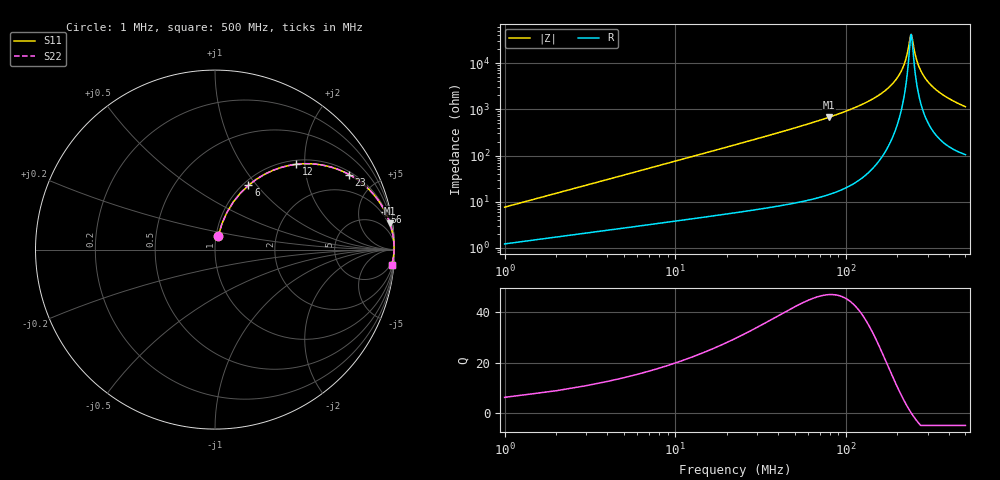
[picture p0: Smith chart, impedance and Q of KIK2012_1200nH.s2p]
!version-2
!date-01.2022
!Series
# MHz S RI R 50
!Freq ReS11 ImS11 ReS21 ImS21 ReS12 ImS12 ReS22 ImS22
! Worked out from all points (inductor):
!   500 points, 1 MHz to 500 MHz, reference 50 ohm
!   read as one part in series: L = 1.2 uH near 3 MHz
!   highest Q = 47 at 79 MHz (marker M1), where L = 1.35 uH
!   self-resonance near 240 MHz
!   S11 on the Smith chart (normalised r, x): 1 MHz: 1.02, +0.15; 6 MHz: 1.06, +0.91; 12 MHz: 1.08, +1.81; 23 MHz: 1.12, +3.50; 56 MHz: 1.20, +8.93; 500 MHz: 3, -23
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1  0.0175 0.0732  0.9825 -0.0732  0.9825 -0.0732  0.0175 0.0732
4  0.1015 0.2647  0.8985 -0.2647  0.8985 -0.2647  0.1015 0.2647
6  0.186 0.3579  0.814 -0.3579  0.814 -0.3579  0.186 0.3579
12  0.454 0.4754  0.546 -0.4754  0.546 -0.4754  0.454 0.4754
23  0.747 0.4183  0.253 -0.4183  0.253 -0.4183  0.747 0.4183
36  0.8787 0.3132  0.1213 -0.3132  0.1213 -0.3132  0.8787 0.3132
56  0.9479 0.2111  0.0521 -0.2111  0.0521 -0.2111  0.9479 0.2111
79  0.9751 0.1455  0.0249 -0.1455  0.0249 -0.1455  0.9751 0.1455
85  0.979 0.1332  0.021 -0.1332  0.021 -0.1332  0.979 0.1332
168  0.9965 0.0402  0.00348 -0.0402  0.00348 -0.0402  0.9965 0.0402
195  0.9975 0.0232  0.00251 -0.0232  0.00251 -0.0232  0.9975 0.0232
214  0.9977 0.0129  0.00229 -0.0129  0.00229 -0.0129  0.9977 0.0129
226  0.9977 0.00687  0.00228 -0.00687  0.00228 -0.00687  0.9977 0.00687
240  0.9976 0.000275  0.00239 -0.000275  0.00239 -0.000275  0.9976 0.000275
243  0.9976 -0.00109  0.00242 0.00109  0.00242 0.00109  0.9976 -0.00109
251  0.9975 -0.00464  0.00254 0.00464  0.00254 0.00464  0.9975 -0.00464
263  0.9972 -0.00976  0.00278 0.00976  0.00278 0.00976  0.9972 -0.00976
280  0.9968 -0.0167  0.00321 0.0167  0.00321 0.0167  0.9968 -0.0167
303  0.996 -0.0254  0.00395 0.0254  0.00395 0.0254  0.996 -0.0254
334  0.9948 -0.0364  0.0052 0.0364  0.0052 0.0364  0.9948 -0.0364
417  0.9903 -0.0625  0.00968 0.0625  0.00968 0.0625  0.9903 -0.0625
500  0.9845 -0.0855  0.0155 0.0855  0.0155 0.0855  0.9845 -0.0855
